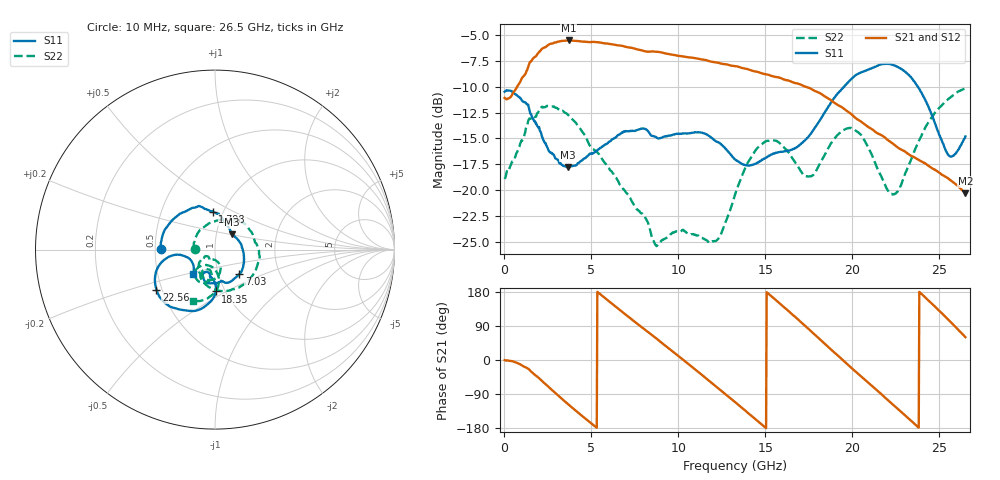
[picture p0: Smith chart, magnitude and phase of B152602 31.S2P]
!  2-Port S-parameters saved by WinCal
! VAR MeasName=S-Parameters (CALIBRATED_DATA) read from VNA (N5242A)
! VAR MeasDate=2016-1-5 16:30:43
! VAR NAME=B152602 31
! VAR FILENAME=B152602 31.S2P
! VAR DATE=2016-1-5 16:30:43
! VAR PHYS_PORTS=1,2
# Hz S DB R 50
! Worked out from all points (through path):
!   801 points, 10 MHz to 26.5 GHz, reference 50 ohm
!   highest |S21| = -5.54 dB at 3.685 GHz (marker M1); lowest = -20.3 dB at 26.5 GHz (marker M2)
!   group delay of S21, straight-line fit = 108 ps
!   lowest |S11| = -17.8 dB at 3.652 GHz (marker M3), VSWR 1.30, Z = 59.6 + j10.5 ohm
!   |S11| at or under -10 dB: start of sweep to 19.53 GHz; 23.77 GHz to end of sweep
!   |S22| runs from -25.4 to -10.1 dB; largest |S21 - S12| = 0.0029
!   S11 on the Smith chart (normalised r, x): 10 MHz: 0.54, +0.00; 1.798 GHz: 0.90, +0.39; 7.03 GHz: 1.26, -0.36; 18.35 GHz: 0.90, -0.45; 22.56 GHz: 0.47, -0.25; 26.5 GHz: 0.76, -0.21
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1e7  -10.49 179.6  -11.08 -0.4  -11.09 -0.3  -18.91 179.3
9.3715e8  -11.17 132.8  -9.42 -12.2  -9.42 -12.2  -15.40 78.3
1.798075e9  -13.57 93.2  -7.06 -41.0  -7.06 -41.0  -12.92 11.0
2.758338e9  -16.51 62.5  -5.83 -80.4  -5.82 -80.4  -11.92 -44.6
3.652375e9  -17.78 41.9  -5.54 -116.4  -5.54 -116.3  -12.71 -83.4
3.685488e9  -17.76 41.1  -5.54 -117.7  -5.54 -117.7  -12.78 -84.6
4.447075e9  -17.14 22.9  -5.64 -147.0  -5.64 -146.9  -14.29 -109.3
5.639125e9  -15.76 -9.8  -5.78 168.7  -5.78 168.7  -17.06 -131.1
7.02985e9  -14.29 -45.2  -6.17 117.5  -6.15 117.6  -20.28 -143.4
8.851038e9  -15.00 -78.3  -6.64 52.5  -6.62 52.4  -25.16 -130.0
1.077156e10  -14.46 -96.6  -7.20 -17.6  -7.17 -17.6  -24.25 -115.4
1.222851e10  -15.33 -112.3  -7.68 -72.1  -7.67 -72.0  -24.80 -89.7
1.3255e10  -17.02 -114.9  -8.02 -110.7  -8.01 -110.9  -20.44 -72.6
1.524175e10  -16.65 -100.8  -8.89 172.3  -8.89 172.4  -15.22 -101.7
1.656625e10  -16.04 -97.1  -9.58 119.6  -9.52 119.7  -16.96 -119.8
1.769208e10  -14.34 -89.5  -10.27 73.0  -10.23 73.2  -18.59 -104.8
1.835432e10  -12.64 -89.0  -10.87 45.2  -10.81 45.3  -16.78 -97.1
2.007618e10  -9.06 -106.3  -12.85 -26.1  -12.83 -26.1  -14.12 -119.7
2.209604e10  -7.81 -137.2  -15.24 -107.9  -15.16 -108.3  -20.16 -118.7
2.255961e10  -8.05 -145.6  -15.80 -126.8  -15.79 -127.2  -20.17 -100.5
2.553974e10  -16.62 -156.9  -18.91 105.4  -18.89 105.4  -11.17 -99.1
2.65e10  -14.80 -132.9  -20.30 60.3  -20.26 60.2  -10.14 -113.6
